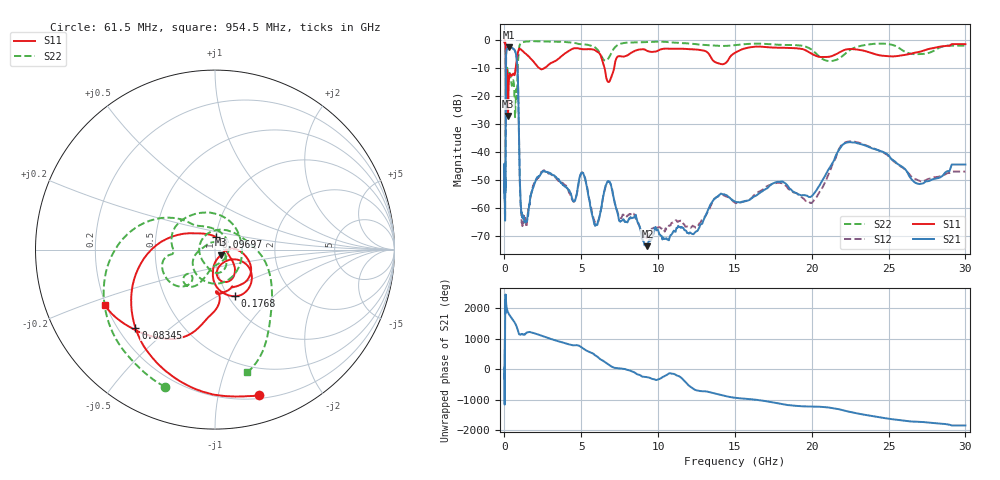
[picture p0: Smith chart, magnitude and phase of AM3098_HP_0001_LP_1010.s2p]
! Date/Time: Thu, Feb 28, 2019 8:32 AM
! Network Analyzer: Agilent Technologies E8364B Rev: A.07.50.67
! Sweep from 0.010 to 30.000 GHz, 1601 Points, Sweep Type: LOG
! Power Supply: 5.022 V, 0.001 A
# Hz S DB R 50
!freq MagS11 AngS11 MagS21 AngS21 MagS12 AngS12 MagS22 AngS22
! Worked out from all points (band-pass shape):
!   1601 points, 10 MHz to 30 GHz, reference 50 ohm
!   highest |S21| = -2.79 dB at 269.1 MHz (marker M1); lowest = -73.5 dB at 9.302 GHz (marker M2)
!   |S21| within 3 dB of the highest: 105.6 MHz to 772 MHz (666.5 MHz wide, 152 % of centre)
!   lowest |S11| = -27.2 dB at 233.9 MHz (marker M3), VSWR 1.09, Z = 53.4 - j3 ohm
!   |S11| at or under -10 dB: 91.06 MHz to 730.5 MHz (639.4 MHz wide, 156 % of centre); 2.222 GHz to 2.65 GHz (427.9 MHz wide, 17.6 % of centre); 6.509 GHz to 7.143 GHz (633.5 MHz wide, 9.28 % of centre)
!   |S22| runs from -27.6 to -0.6 dB; largest |S21 - S12| = 0.011
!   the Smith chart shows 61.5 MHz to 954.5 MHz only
!   S11 on the Smith chart (normalised r, x): 61.5 MHz: 0.23, -1.32; 83.45 MHz: 0.27, -0.38; 96.97 MHz: 1.00, +0.14; 176.8 MHz: 1.08, -0.61; 954.5 MHz: 0.19, -0.23
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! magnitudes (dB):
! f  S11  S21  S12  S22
! 10 MHz  -0.3  -44.2  -45.6  -0.6
! 38.04 MHz  -0.5  -58.5  -59.6  -1.0
! 61.5 MHz  -1.4  -52.2  -53.8  -1.8
! 83.45 MHz  -4.1  -31.2  -31.0  -4.6
! 96.97 MHz  -23.1  -9.0  -9.0  -22.6
! 144.7 MHz  -14.7  -3.5  -3.4  -12.8
! 176.8 MHz  -11.0  -3.3  -3.3  -10.0
! 233.9 MHz  -27.2  -2.9  -2.8  -12.5
! 269.1 MHz  -16.9  -2.8  -2.8  -12.7
! 550.5 MHz  -12.2  -3.3  -3.2  -14.5
! 825.6 MHz  -6.3  -8.5  -8.5  -17.9
! 954.5 MHz  -3.3  -37.3  -37.4  -3.0
! 1.154 GHz  -3.9  -62.9  -65.2  -1.0
! 2.084 GHz  -9.2  -49.4  -49.7  -0.6
! 5.077 GHz  -3.4  -47.4  -47.3  -1.7
! 5.929 GHz  -3.9  -65.7  -65.0  -3.0
! 6.753 GHz  -15.1  -50.3  -50.4  -6.8
! 7.926 GHz  -5.8  -64.9  -62.5  -1.1
! 9.302 GHz  -4.1  -73.5  -70.1  -0.9
! 19.9 GHz  -4.8  -56.0  -58.1  -3.3
! 22.67 GHz  -3.4  -36.6  -36.3  -3.2
! 30 GHz  -1.6  -44.5  -46.9  -2.2
